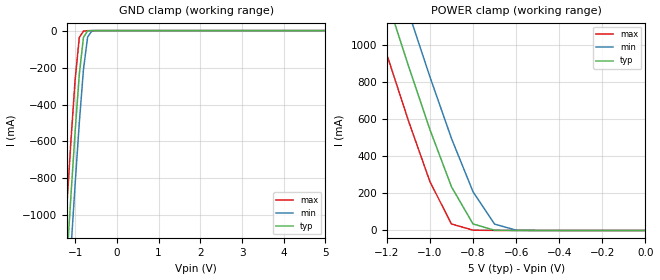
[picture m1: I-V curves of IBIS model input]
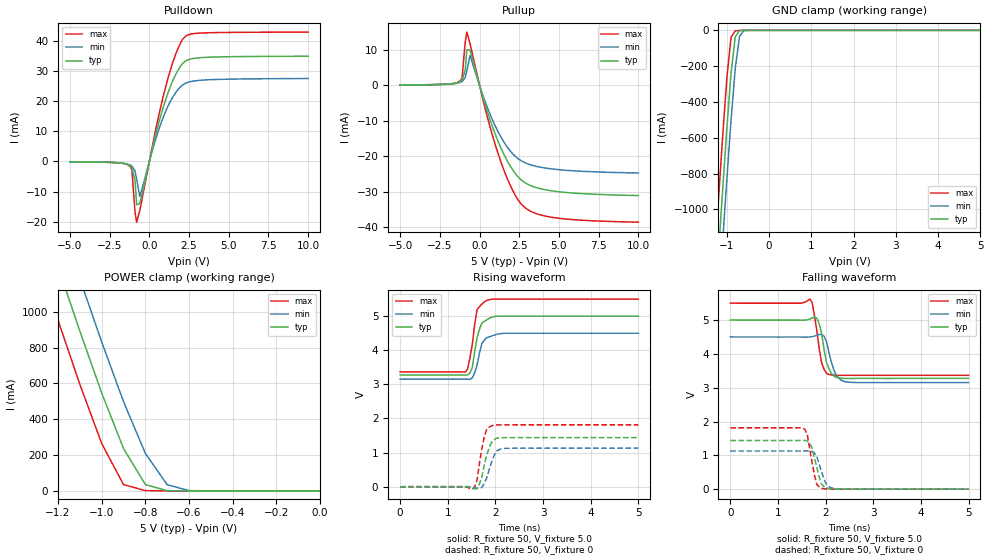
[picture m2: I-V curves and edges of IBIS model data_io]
| SOJ package &   Industrial  Operation
[IBIS Ver]   3.2
[Comment Char]   |_char
[File name]   as7c1024b_soji.ibs
[File Rev]   1.0
[Date]   Jun 9, 2004 2:43:45 PM
[Source]
Alliance Semiconductor Corporation
[Notes]
This model  is for SOJ package &
 Industrial  Operation
[Disclaimer]
Data is for modeling purpose only and is not guaranted.
This IBIS model is provided on an "AS IS" basis and Alliance Semiconductor makes
absolutely no warranty with respect to the information contained
herein.The entire risk as to quality and performance
is with the Customer. ACCORDINGLY, IN NO EVENT SHALL THE COMPANY BE
LIABLE FOR ANY DAMAGES, WHETHER IN CONTRACT OR TORT,INCLUDING ANY
LOST PROFITS OR OTHER INCIDENTAL, CONSEQUENTIAL, EXEMPLARY, OR
PUNITIVE DAMAGES ARISING OUT OF THE USE OR APPLICATION OF THE IBIS
model provided in this package.
[Copyright]
Alliance Semiconductor Corporation
| SOJ Package & Industrial Operation.
[Component]   AS7C1024B_SOJI
Si_location Pin
Timing_location Pin
[Manufacturer]   Alliance Semiconductor Corporation
[Package]
R_pkg   351.65m   239.7m   463.6m
L_pkg   8.523nH   5.387nH   11.66nH
C_pkg   1.885pF   1.215pF   2.556pF
[Pin] signal_name   model_name
1   NC   NC
2   A16   input
3   A14   input
4   A12   input
5   A7   input
6   A6   input
7   A5   input
8   A4   input
9   A3   input
10   A2   input
11   A1   input
12   A0   input
13   IO0   data_io
14   IO1   data_io
15   IO2   data_io
16   GND   GND
17   IO3   data_io
18   IO4   data_io
19   IO5   data_io
20   IO6   data_io
21   IO7   data_io
22   NCE1   input
23   A10   input
24   NOE   input
25   A11   input
26   A9   input
27   A8   input
28   A13   input
29   NWE   input
30   CE2   input
31   A15   input
32   VCC   POWER
| Models and submodels in the file (2): input (Input), data_io (I/O)
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[Model]   input
Model_type Input
Vinh=2.2V
Vinl=0.8V
C_comp   4pF   4pF   4pF
[Model Spec]
[Temperature Range] 25   85   -40
[Voltage Range]   5.0   4.5   5.5
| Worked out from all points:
|   GND clamp passes 1 mA (typ) near -0.67 V on its own axis
|   POWER clamp passes 1 mA (typ) near -0.68 V on its own axis
[GND Clamp]
-5V       -16.01A    -16.28A    -15.75A
-1.3V     -1.622A    -1.916A    -1.322A
-1.2V     -1.253A    -1.547A    -953.4mA
-1.1V     -892.6mA   -1.184A    -596mA
-1V       -547.3mA   -832.1mA   -266.1mA
-900mV    -237.4mA   -499.3mA   -37.66mA
-800mV    -36.26mA   -209.9mA   -2.709mA
-700mV    -1.383mA   -34.75mA   -458.6uA
-600mV    -81.45uA   -1.835mA   -48.66uA
5V        292.5pA    86.47uA    -195.3pA
[POWER Clamp]
-5V       16.01A     16.27A     15.75A
-1.3V     1.621A     1.915A     1.322A
-1.2V     1.252A     1.546A     952.5mA
-1.1V     891.7mA    1.183A     594.7mA
-1V       546.1mA    831.3mA    264.7mA
-900mV    236.6mA    498.2mA    35.19mA
-800mV    35.4mA     209.4mA    1.73mA
-700mV    1.248mA    34.46mA    445.9uA
-600mV    85.03uA    1.813mA    86.82uA
0V        292.5pA    2.095nA    135pA
[Model]   data_io
Model_type I/O
Enable Active-High
Polarity Non-Inverting
Vinh=2.2V
Vinl=0.8V
Vref=1.728V
Vmeas=1.5V
Rref=168
Cref=30pF
C_comp   4pF   4pF   4pF
[Temperature Range] 25   85   -40
[Voltage Range]   5.0   4.5   5.5
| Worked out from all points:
|   slope of the pulldown table from 0 to 0.75 V, typ, clamps not added: 47.5 ohm
|   slope of the pullup table from 0 to 0.75 V, typ, clamps not added: 69.3 ohm
|   GND clamp passes 1 mA (typ) near -0.67 V on its own axis
|   POWER clamp passes 1 mA (typ) near -0.68 V on its own axis
|   falling waveform, R_fixture 50, V_fixture 5.0: 20-80 % time 149ps typ, 165ps min, 137ps max; typ from 5 V to 3.27 V
|   falling waveform, R_fixture 50, V_fixture 0: 20-80 % time 154ps typ, 162ps min, 139ps max; typ from 1.44 V to 0.003 V
|   rising waveform, R_fixture 50, V_fixture 5.0: 20-80 % time 148ps typ, 150ps min, 134ps max; typ from 3.27 V to 5 V
|   rising waveform, R_fixture 50, V_fixture 0: 20-80 % time 158ps typ, 162ps min, 134ps max; typ from 0 V to 1.44 V
[Pullup]
-5V       90uA       90uA       90uA
-1.2V     1.068mA    839uA      1.331mA
-1.1V     1.45mA     1.063mA    2.038mA
-900mV    4.251mA    2.175mA    12.13mA
-800mV    9.897mA    4.005mA    14.96mA
-600mV    9.913mA    8.355mA    11.77mA
300mV     -4.636mA   -3.916mA   -5.565mA
1.1V      -15.02mA   -12.47mA   -18.29mA
1.8V      -21.7mA    -17.71mA   -26.79mA
2.6V      -26.53mA   -21.16mA   -33.26mA
4.5V      -29.66mA   -23.5mA    -37.1mA
10V       -31.02mA   -24.68mA   -38.51mA
[Pulldown]
-5V       -120uA     -120uA     -100uA
-1.2V     -1.484mA   -1.15mA    -1.731mA
-1.1V     -2.045mA   -1.499mA   -2.745mA
-900mV    -6.312mA   -3.157mA   -16.92mA
-800mV    -14.39mA   -5.87mA    -20.17mA
-600mV    -13.97mA   -11.66mA   -16.24mA
300mV     6.815mA    5.674mA    8.013mA
900mV     18.45mA    15.03mA    22.16mA
1.5V      27.11mA    21.62mA    33.26mA
2.1V      32.56mA    25.44mA    40.62mA
3.2V      34.48mA    26.97mA    42.65mA
10V       34.96mA    27.56mA    42.98mA
[GND Clamp]
-5V       -16.01A    -16.28A    -15.75A
-1.3V     -1.622A    -1.916A    -1.322A
-1.2V     -1.253A    -1.547A    -953.4mA
-1.1V     -892.6mA   -1.184A    -596mA
-1V       -547.3mA   -832.1mA   -266.1mA
-900mV    -237.4mA   -499.3mA   -37.66mA
-800mV    -36.26mA   -209.9mA   -2.709mA
-700mV    -1.383mA   -34.75mA   -458.6uA
-600mV    -81.45uA   -1.835mA   -48.66uA
5V        292.5pA    86.47uA    -195.3pA
[POWER Clamp]
-5V       16.01A     16.27A     15.75A
-1.3V     1.621A     1.915A     1.322A
-1.2V     1.252A     1.546A     952.5mA
-1.1V     891.7mA    1.183A     594.7mA
-1V       546.1mA    831.3mA    264.7mA
-900mV    236.6mA    498.2mA    35.19mA
-800mV    35.4mA     209.4mA    1.73mA
-700mV    1.248mA    34.46mA    445.9uA
-600mV    85.03uA    1.813mA    86.82uA
0V        292.5pA    2.095nA    135pA
[Falling Waveform]
R_fixture=50
V_fixture=5.0
V_fixture_min=4.5
V_fixture_max=5.5
0s        5V         4.5V       5.5V
1.667ns   5.029V     4.499V     5.619V
1.717ns   5.056V     4.507V     5.519V
1.869ns   4.875V     4.576V     4.122V
1.919ns   4.586V     4.572V     3.717V
2.02ns    3.751V     4.357V     3.422V
2.071ns   3.564V     4.039V     3.394V
2.222ns   3.305V     3.368V     3.368V
2.424ns   3.272V     3.171V     3.366V
5ns       3.274V     3.152V     3.366V
[Falling Waveform]
R_fixture=50
V_fixture=0
V_fixture_min=0
V_fixture_max=0
0s        1.438V     1.129V     1.814V
1.566ns   1.443V     1.132V     1.769V
1.616ns   1.423V     1.133V     1.61V
1.717ns   1.215V     1.117V     789.7mV
1.768ns   921.2mV    1.067V     402.8mV
1.818ns   629.7mV    952.1mV    133mV
1.919ns   140.9mV    502.4mV    27.71mV
2.02ns    35.44mV    139.6mV    6.629mV
2.222ns   4.781mV    18.08mV    2.79mV
5ns       2.726mV    2.728mV    2.77mV
[Rising Waveform]
R_fixture=50
V_fixture=5.0
V_fixture_min=4.5
V_fixture_max=5.5
0s        3.275V     3.153V     3.365V
1.364ns   3.27V      3.152V     3.356V
1.414ns   3.28V      3.15V      3.441V
1.515ns   3.5V       3.189V     4.17V
1.566ns   3.969V     3.344V     4.763V
1.616ns   4.368V     3.565V     5.193V
1.717ns   4.8V       4.196V     5.353V
1.818ns   4.889V     4.368V     5.46V
2.222ns   4.997V     4.496V     5.497V
5ns       4.997V     4.497V     5.497V
[Rising Waveform]
R_fixture=50
V_fixture=0
V_fixture_min=0
V_fixture_max=0
0s        0V         735.4nV    0V
1.515ns   -25.33mV   -4.031mV   -70.19mV
1.616ns   -49.61mV   -46.56mV   209.8mV
1.667ns   92.94mV    -53.32mV   699.6mV
1.717ns   301.9mV    -17.12mV   1.135V
1.818ns   931.5mV    263.3mV    1.694V
1.919ns   1.3V       715.8mV    1.786V
2.02ns    1.423V     1.04V      1.813V
2.172ns   1.437V     1.121V     1.812V
5ns       1.44V      1.13V      1.815V
[Ramp]
R_load=50
dV/dt_r   8.639E-1/1.562E-10   6.781E-1/1.584E-10   1.089E+0/1.338E-10
dV/dt_f   1.035E+0/1.438E-10   8.087E-1/1.555E-10   1.281E+0/1.259E-10
|[End   data_io
